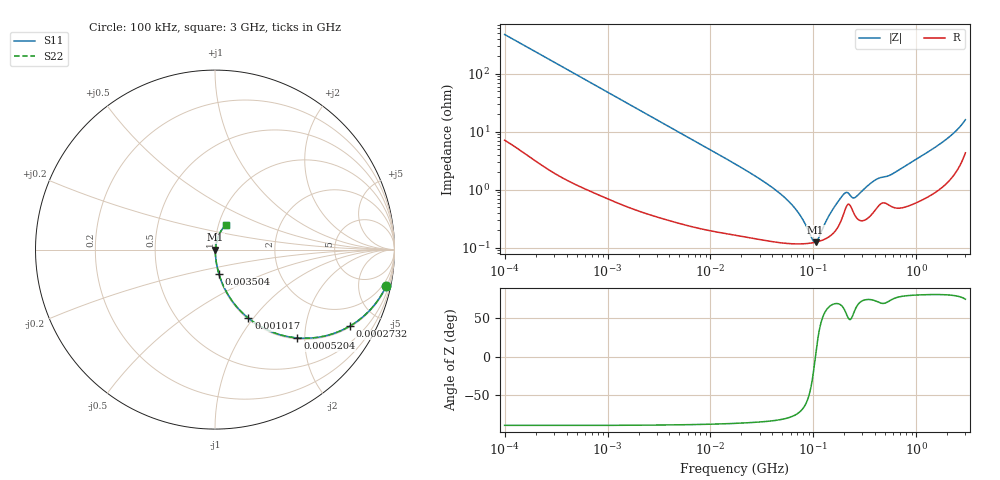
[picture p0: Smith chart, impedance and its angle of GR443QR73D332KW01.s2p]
!Murata Part Number: GR443QR73D332KW01
!These Parameters are Measured in Series Mode Connection
!Data Generated on Mar 13, 2026
!  o--ll--o
!Port1  Port2
!  o------o
!Operation Temp=25[degC], DC Bias Voltage=0[V]
!Freq. Start=100[kHz] Stop=3[GHz] 401[Steps]
# Hz S RI R 50
!Freq.(Hz) S11(Real) S11(Imag) S21(Real) S21(Imag) S12(Real) S12(Imag) S22(Real) S22(Imag)
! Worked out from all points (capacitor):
!   401 points, 100 kHz to 3 GHz, reference 50 ohm
!   read as one part in series: C = 3.36 nF near 105.3 kHz
!   lowest |Z| = 125 mohm at 105.2 MHz (marker M1)
!   series resonance near 104.7 MHz, so ESL is about 690 pH
!   S11 on the Smith chart (normalised r, x): 100 kHz: 1.14, -9.45; 273.2 kHz: 1.04, -3.49; 520.4 kHz: 1.02, -1.84; 1.017 MHz: 1.01, -0.95; 3.504 MHz: 1.01, -0.28; 3 GHz: 1.09, +0.31
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100000  0.9544 -0.2012  0.0456 0.2012  0.0456 0.2012  0.9544 -0.2012
171810  0.8812 -0.3168  0.1188 0.3168  0.1188 0.3168  0.8812 -0.3168
273224  0.7503 -0.4267  0.2497 0.4267  0.2497 0.4267  0.7503 -0.4267
520403  0.4589 -0.492  0.5411 0.492  0.5411 0.492  0.4589 -0.492
562235  0.4216 -0.4874  0.5784 0.4874  0.5784 0.4874  0.4216 -0.4874
1017073  0.1863 -0.3821  0.8137 0.3821  0.8137 0.3821  0.1863 -0.3821
3161081  0.0261 -0.1489  0.9739 0.1489  0.9739 0.1489  0.0261 -0.1489
3504345  0.0218 -0.135  0.9782 0.135  0.9782 0.135  0.0218 -0.135
1.77727e7  0.00236 -0.027  0.9976 0.027  0.9976 0.027  0.00236 -0.027
3.657227e7  0.00145 -0.0121  0.9985 0.0121  0.9985 0.0121  0.00145 -0.0121
5.667996e7  0.00122 -0.00636  0.9988 0.00636  0.9988 0.00636  0.00122 -0.00636
7.525761e7  0.00118 -0.00331  0.9988 0.00331  0.9988 0.00331  0.00118 -0.00331
9.738194e7  0.00121 -0.000724  0.9988 0.000724  0.9988 0.000724  0.00121 -0.000724
1.0521e8  0.00125 4.9e-05  0.9988 -4.9e-05  0.9988 -4.9e-05  0.00125 4.9e-05
1.470833e8  0.00163 0.00364  0.9984 -0.00364  0.9984 -0.00364  0.00163 0.00364
1.952919e8  0.00372 0.0073  0.9963 -0.0073  0.9963 -0.0073  0.00372 0.0073
2.109903e8  0.00529 0.00722  0.9947 -0.00722  0.9947 -0.00722  0.00529 0.00722
2.52704e8  0.00368 0.00628  0.9963 -0.00628  0.9963 -0.00628  0.00368 0.00628
3.916425e8  0.00443 0.0136  0.9956 -0.0136  0.9956 -0.0136  0.00443 0.0136
5.475153e8  0.00562 0.0166  0.9944 -0.0166  0.9944 -0.0166  0.00562 0.0166
1.746113e9  0.0143 0.0611  0.9857 -0.0611  0.9857 -0.0611  0.0143 0.0611
3e9  0.0621 0.1393  0.9379 -0.1393  0.9379 -0.1393  0.0621 0.1393
